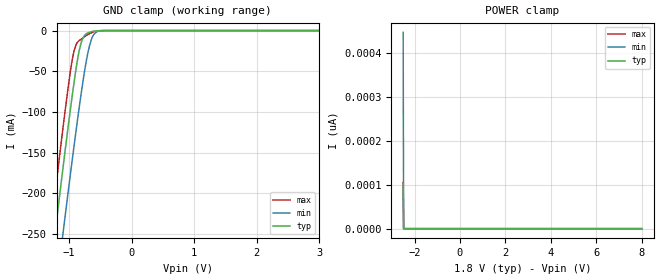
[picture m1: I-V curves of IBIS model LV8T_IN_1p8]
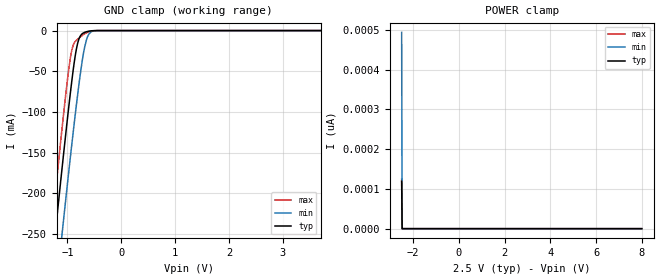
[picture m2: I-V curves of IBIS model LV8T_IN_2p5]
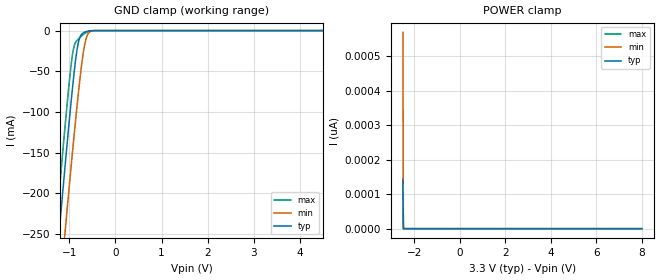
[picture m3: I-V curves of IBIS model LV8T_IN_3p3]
| TEXAS INSTRUMENTS INCORPORATED
| Analog Signal Chain - Interface - Logic
| IBIS Model of SN74LV8T165
| Parallel-Load 8-Bit Shift Registers
| TSSOP 20-pin (PW) and WQFN 20-pin (BQB) Packages
[IBIS Ver]   3.2
[Comment Char]  |_char
[File Name]   sn74lv8t165.ibs
[File Rev]   1.0
[Date]   11/2023
[Source]   Data created from SPICE simulations at TI.
[Notes]   The following is an IBIS list for the LV8T165.
|   Enable is active HIGH
|   This model produces multiple non-monotonicity warnings. These are
|   expected and accurately represent the operation of the device.
[Disclaimer] Property of Texas Instruments Incorporated.  Unauthorized
   reproduction and/or distribution is strictly prohibited.
   This product is protected under copyright law.
   Created 2023, (C) Copyright 2023, Texas Instruments Inc.,
   All Rights Reserved.
   UNLESS THERE IS A SIGNED, WRITTEN AGREEMENT TO THE
   CONTRARY, TEXAS INSTRUMENTS () IS PROVIDING THE IBIS
   MODELS  AND WITHOUT ANY WARRANTY, EXPRESSED OR
   IMPLIED.  TI assumes no liability for:
   1) the accuracy of the IBIS models provided to your
   company;
   2) the proper functioning of these IBIS Models in your
   design or for any resulting applications; or
   3) infringement of patents, copyrights or intellectual
   property rights resulting from your use of these IBIS
   models.
   TI provides IBIS Models as a service to our customers.
   You and your company shall not distribute, sell or give
   these models to anyone else without prior written
   permission from TI.
   TI reserves the right to make changes to our products or
   to discontinue any semiconductor product or service
   without notice, and advises our customers to obtain the
   latest version of relevant information to verify, before
   placing orders, that the information being relied on is
   current.
   Please be aware that your receipt and use of the IBIS
   information provided shall serve as acceptance of these
   terms and conditions.  If you do not accept these terms,
   you should return or destroy the IBIS models and any
   other accompanying information immediately.
[Component]   SN74LV8T165BQB
[Manufacturer]   TI
[Package]   |WQFN, 16 pin BQB
|   typ   min   max
R_pkg   0.05   0.04   0.06
L_pkg   1.0nH   0.8nH   1.2nH
C_pkg   0.2pF   0.16pF   0.24pF
[Pin]   signal_name   model_name   R_pin  L_pin  C_pin
1   SH_LDN   LV8T_IN   NA   NA   NA
2   CLK   LV8T_IN   NA   NA   NA
3   E   LV8T_IN   NA   NA   NA
4   F   LV8T_IN   NA   NA   NA
5   G   LV8T_IN   NA   NA   NA
6   H   LV8T_IN   NA   NA   NA
7   Q_HN   LV8T_OUT   NA   NA   NA
8   GND   GND   NA   NA   NA
9   Q_H   LV8T_OUT   NA   NA   NA
10   SER   LV8T_IN   NA   NA   NA
11   A   LV8T_IN   NA   NA   NA
12   B   LV8T_IN   NA   NA   NA
13   C   LV8T_IN   NA   NA   NA
14   D   LV8T_IN   NA   NA   NA
15   CLK_INH   LV8T_IN   NA   NA   NA
16   VCC   POWER   NA   NA   NA
[Component]   SN74LV8T165PW
[Manufacturer]   TI
[Package]   |TSSOP, 16 pin PW
|   typ   min   max
R_pkg   0.05   0.04   0.06
L_pkg   1.0nH   0.8nH   1.2nH
C_pkg   0.2pF   0.16pF   0.24pF
[Pin]   signal_name   model_name   R_pin  L_pin  C_pin
1   SH_LDN   LV8T_IN   NA   NA   NA
2   CLK   LV8T_IN   NA   NA   NA
3   E   LV8T_IN   NA   NA   NA
4   F   LV8T_IN   NA   NA   NA
5   G   LV8T_IN   NA   NA   NA
6   H   LV8T_IN   NA   NA   NA
7   Q_HN   LV8T_OUT   NA   NA   NA
8   GND   GND   NA   NA   NA
9   Q_H   LV8T_OUT   NA   NA   NA
10   SER   LV8T_IN   NA   NA   NA
11   A   LV8T_IN   NA   NA   NA
12   B   LV8T_IN   NA   NA   NA
13   C   LV8T_IN   NA   NA   NA
14   D   LV8T_IN   NA   NA   NA
15   CLK_INH   LV8T_IN   NA   NA   NA
16   VCC   POWER   NA   NA   NA
|   Model Selector
[Model Selector]   LV8T_IN
LV8T_IN_1p8   1.8-V Vcc Input Model
LV8T_IN_2p5   2.5-V Vcc Input Model
LV8T_IN_3p3   3.3-V Vcc Input Model
LV8T_IN_5   5.0-V Vcc Input Model
[Model Selector]   LV8T_OUT
LV8T_OUT_1p8   1.8-V Vcc Output Model
LV8T_OUT_2p5   2.5-V Vcc Output Model
LV8T_OUT_3p3   3.3-V Vcc Output Model
LV8T_OUT_5   5.0-V Vcc Output Model
| Models and submodels in the file (8): LV8T_IN_1p8 (Input), LV8T_IN_2p5 (Input), LV8T_IN_3p3 (Input), LV8T_IN_5 (Input), LV8T_OUT_1p8 (3-state), LV8T_OUT_2p5 (3-state), LV8T_OUT_3p3 (3-state), LV8T_OUT_5 (3-state)
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|   Model LV8T_IN_33
[Model]   LV8T_IN_1p8
Model_type   Input
Vinl = 0.51
Vinh = 1.1
|   typ   min   max
C_comp   0.94pF   0.94pF   0.94pF
[Voltage Range]   1.8   1.65   1.95
[Temperature Range]   27   125   -40
[Power Clamp Reference]   1.8   1.65   1.95
[GND Clamp Reference]   0   0   0
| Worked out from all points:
|   GND clamp passes 1 mA (typ) near -0.62 V on its own axis
[GND Clamp]
|   Voltage   I(typ)   I(min)   I(max)
-2.5V     -1.102A    -1.155A    -1.067A
-1.292V   -294.1mA   -373.9mA   -246.2mA
-1.188V   -226.4mA   -306.9mA   -177.6mA
-1.083V   -160.1mA   -240.9mA   -111mA
-967mV    -90.42mA   -170.1mA   -44.5mA
-914.5mV  -60.98mA   -138.9mA   -23.57mA
-809.5mV  -15.97mA   -79.55mA   -10.72mA
-757mV    -6.46mA    -52.6mA    -7.795mA
-673mV    -2.071mA   -18.84mA   -3.804mA
-599.5mV  -718.5uA   -4.334mA   -1.428mA
-442mV    -12.39uA   -73.17uA   -11.72uA
8V        0A         0A         0A
[POWER Clamp]
|   Voltage   I(typ)   I(min)   I(max)
-2.5V     102.3pA    446.2pA    104.8pA
-2.479V   0A         0A         0A
-2.469V   0A         0A         0A
8V        0A         0A         0A
[Model]   LV8T_IN_2p5
Model_type   Input
Vinl = 0.65
Vinh = 1.28
|   typ   min   max
C_comp   0.94pF   0.94pF   0.94pF
[Voltage Range]   2.5   2.25   2.75
[Temperature Range]   27   125   -40
[Power Clamp Reference]   2.5   2.25   2.75
[GND Clamp Reference]   0   0   0
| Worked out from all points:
|   GND clamp passes 1 mA (typ) near -0.62 V on its own axis
[GND Clamp]
|   Voltage   I(typ)   I(min)   I(max)
-2.5V     -1.102A    -1.155A    -1.067A
-1.292V   -294.1mA   -373.9mA   -246.2mA
-1.188V   -226.4mA   -306.9mA   -177.6mA
-1.083V   -160.1mA   -240.9mA   -111mA
-967mV    -90.42mA   -170.1mA   -44.5mA
-914.5mV  -60.98mA   -138.9mA   -23.57mA
-809.5mV  -15.97mA   -79.55mA   -10.72mA
-757mV    -6.46mA    -52.6mA    -7.795mA
-673mV    -2.071mA   -18.84mA   -3.804mA
-599.5mV  -718.5uA   -4.334mA   -1.428mA
-442mV    -12.39uA   -73.17uA   -11.72uA
8V        0A         0A         0A
[POWER Clamp]
|   Voltage   I(typ)   I(min)   I(max)
-2.5V     119.1pA    493.5pA    124.1pA
-2.479V   0A         0A         0A
-2.469V   0A         0A         0A
8V        0A         0A         0A
[Model]   LV8T_IN_3p3
Model_type   Input
Vinl = 0.75
Vinh = 1.45
|   typ   min   max
C_comp   0.94pF   0.94pF   0.94pF
[Voltage Range]   3.3   3   3.6
[Temperature Range]   27   125   -40
[Power Clamp Reference]   3.3   3   3.6
[GND Clamp Reference]   0   0   0
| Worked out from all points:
|   GND clamp passes 1 mA (typ) near -0.62 V on its own axis
[GND Clamp]
|   Voltage   I(typ)   I(min)   I(max)
-2.5V     -1.102A    -1.155A    -1.067A
-1.292V   -294.1mA   -373.9mA   -246.2mA
-1.188V   -226.4mA   -306.9mA   -177.6mA
-1.083V   -160.1mA   -240.9mA   -111mA
-967mV    -90.42mA   -170.1mA   -44.5mA
-914.5mV  -60.98mA   -138.9mA   -23.57mA
-809.5mV  -15.97mA   -79.55mA   -10.72mA
-757mV    -6.46mA    -52.6mA    -7.795mA
-673mV    -2.071mA   -18.84mA   -3.804mA
-599.5mV  -718.5uA   -4.334mA   -1.428mA
-442mV    -12.39uA   -73.17uA   -11.72uA
8V        0A         0A         0A
[POWER Clamp]
|   Voltage   I(typ)   I(min)   I(max)
-2.5V     139pA      568.9pA    145.5pA
-2.479V   0A         0A         0A
-2.469V   0A         0A         0A
8V        0A         0A         0A
